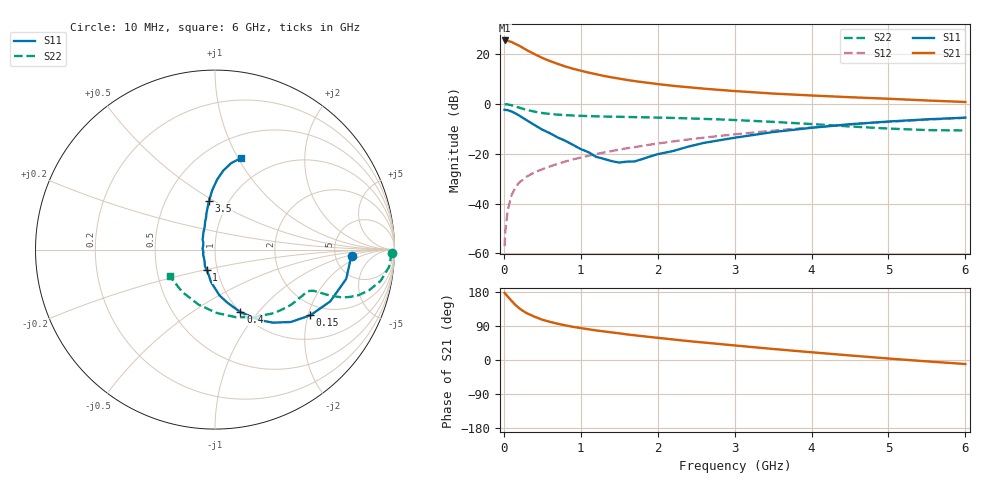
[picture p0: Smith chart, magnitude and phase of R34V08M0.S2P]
! SIEMENS Small Signal Semiconductors
! BFR181
! Si NPN RF Bipolar Junction Transistor in SOT23
! VCE = 4 V  IC = 8 mA
! Common Emitter S-Parameters:  May  1996
# GHz  S  MA  R  50
!  f  S11  S21  S12  S22
! GHz  MAG  ANG  MAG  ANG  MAG  ANG  MAG  ANG
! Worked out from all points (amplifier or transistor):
!   36 points, 10 MHz to 6 GHz, reference 50 ohm
!   highest |S21| = 25.4 dB at 10 MHz (marker M1)
!   |S21| within 3 dB of that: start of sweep to 249.6 MHz
!   unconditionally stable (mu >= 1): 891.9 MHz to 2.741 GHz
!   at 250 MHz: K = 0.54, MSG = 26.4 dB, |S12| = -30.4 dB
!   at 1.4 GHz: K = 1.05, MAG = 13.4 dB, |S12| = -18.9 dB
!   at 6 GHz: K = 0.86, MSG = 3.2 dB, |S12| = -5.6 dB
!   S11 on the Smith chart (normalised r, x): 10 MHz: 7.24, -1.15; 150 MHz: 1.65, -2.07; 400 MHz: 1.00, -0.81; 1 GHz: 0.89, -0.21; 3.5 GHz: 0.81, +0.47; 6 GHz: 0.72, +1.03
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0.01  0.7627 -2.5  18.71 177.2  0.0014 94.4  0.9872 -1.0
0.02  0.7558 -4.9  18.33 174.6  0.0029 85.9  0.9816 -2.3
0.05  0.749 -12.6  18.32 167.5  0.0073 83.9  0.9752 -5.6
0.1  0.704 -24.2  17.46 156.2  0.0147 79.1  0.939 -10.7
0.15  0.645 -34.6  15.97 145.3  0.0209 73.8  0.8891 -14.7
0.2  0.5839 -43.7  14.68 136.8  0.0265 71.0  0.8398 -17.6
0.25  0.5201 -51.5  13.24 129.3  0.0302 68.9  0.7948 -19.4
0.3  0.4667 -57.5  11.95 123.3  0.0351 68.5  0.7564 -20.6
0.4  0.3759 -67.9  9.943 114.2  0.0422 66.7  0.6975 -21.7
0.5  0.304 -76.8  8.342 106.3  0.0489 67.1  0.6555 -22.1
0.6  0.2576 -84.3  7.23 100.7  0.0558 67.2  0.6275 -22.3
0.7  0.212 -90.7  6.344 95.7  0.0627 67.7  0.6086 -22.5
0.8  0.1816 -97.1  5.626 91.4  0.07 67.9  0.5953 -22.7
1  0.124 -111.7  4.629 84.2  0.0837 68.2  0.5757 -23.6
1.1  0.1077 -121.5  4.25 81.1  0.091 68.6  0.5693 -24.2
1.3  0.079 -140.5  3.64 75.5  0.1059 68.2  0.5581 -25.7
1.6  0.0695 174.7  3.02 67.6  0.1287 67.3  0.5467 -28.7
2.2  0.1135 124.9  2.303 54.2  0.1764 64.7  0.5226 -36.2
3.5  0.2725 97.1  1.61 29.1  0.2907 54.5  0.436 -59.5
4.5  0.3912 88.2  1.361 12.0  0.388 43.8  0.3526 -88.7
5.5  0.4902 79.4  1.17 -3.6  0.4819 31.2  0.2981 -127.7
6  0.5293 74.3  1.091 -10.6  0.5247 24.2  0.2925 -149.5
